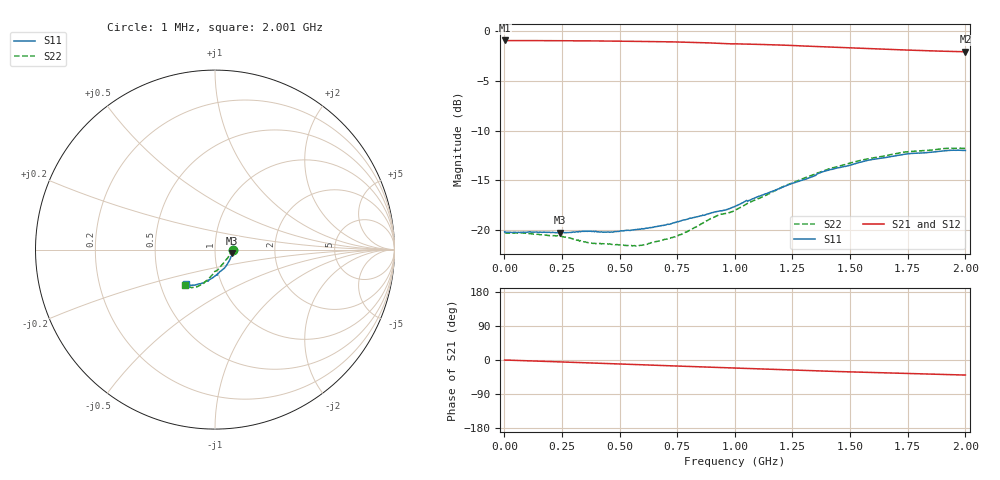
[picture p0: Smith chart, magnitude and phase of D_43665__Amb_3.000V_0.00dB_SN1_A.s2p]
! device id: 43665_
! dir: \\malibu\benchdata\1_engineers\tn_data\43665_75ohm\new\sparar\43665_\amb\3p000v\0p00db
! Serial: 1
! Insertion: A
! Temp: Amb
! VDD: 3.000V
! Attenuation Step: 0.00dB
! IDD: 1.454652e+00mA
! FILE NAME
! DATE 03-27-2009 08:33:22
! CORRECTED  DATA
#  Hz  S  RI  R  75
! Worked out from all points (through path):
!   401 points, 1 MHz to 2.001 GHz, reference 75 ohm
!   highest |S21| = -0.95 dB at 1 MHz (marker M1); lowest = -2.1 dB at 2.001 GHz (marker M2)
!   group delay of S21, straight-line fit = 56.5 ps
!   lowest |S11| = -20.3 dB at 241 MHz (marker M3), VSWR 1.21, Z = 90.7 - j3.66 ohm
!   |S11| at or under -10 dB: start of sweep to end of sweep
!   |S22| runs from -21.6 to -11.8 dB; largest |S21 - S12| = 0.0053
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1000000  0.0983 -0.00166  0.8965 -0.00159  0.8964 -0.00157  0.0978 -0.00128
2.41e8  0.0949 -0.02  0.8904 -0.0776  0.8906 -0.0777  0.0909 -0.02
3.36e8  0.094 -0.0299  0.8861 -0.1085  0.8863 -0.1082  0.0835 -0.0283
3.76e8  0.0927 -0.0343  0.8838 -0.121  0.884 -0.1209  0.0798 -0.0327
4.61e8  0.0872 -0.0443  0.878 -0.1488  0.8782 -0.1488  0.0734 -0.0433
5.71e8  0.0806 -0.0603  0.8677 -0.1846  0.8677 -0.1842  0.0599 -0.0576
6.11e8  0.0772 -0.0666  0.8638 -0.197  0.8638 -0.1967  0.0557 -0.0639
6.71e8  0.0712 -0.077  0.8575 -0.2165  0.8574 -0.2159  0.0488 -0.0736
7.61e8  0.0604 -0.0931  0.8455 -0.2456  0.8457 -0.2448  0.0359 -0.0879
9.16e8  0.0321 -0.1194  0.817 -0.2934  0.8178 -0.2922  0.0105 -0.1167
9.66e8  0.0257 -0.1243  0.8078 -0.3035  0.8087 -0.3022  -0.00089 -0.1217
1.001e9  0.0208 -0.1301  0.8035 -0.312  0.8047 -0.311  -0.00546 -0.1257
1.041e9  0.0118 -0.1384  0.7974 -0.3236  0.7987 -0.323  -0.00938 -0.1329
1.211e9  -0.0237 -0.1634  0.7653 -0.3687  0.7671 -0.3687  -0.0341 -0.162
1.336e9  -0.0525 -0.178  0.7383 -0.396  0.74 -0.3963  -0.0558 -0.1805
1.366e9  -0.0623 -0.1831  0.7317 -0.4031  0.7328 -0.4052  -0.0605 -0.1855
1.406e9  -0.0711 -0.1869  0.7224 -0.4117  0.7233 -0.4143  -0.0668 -0.1914
1.541e9  -0.1006 -0.1945  0.694 -0.4351  0.6939 -0.4385  -0.0924 -0.2033
1.671e9  -0.1236 -0.1981  0.6673 -0.4564  0.6654 -0.4598  -0.1154 -0.209
1.751e9  -0.1362 -0.1995  0.6512 -0.4684  0.6492 -0.4718  -0.1289 -0.2117
1.911e9  -0.1542 -0.1973  0.6209 -0.4904  0.6181 -0.491  -0.1555 -0.2044
2.001e9  -0.1597 -0.194  0.6052 -0.5027  0.6001 -0.5044  -0.1664 -0.196
